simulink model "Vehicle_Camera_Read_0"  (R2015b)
settings: Solver=FixedStepDiscrete  StartTime=0.0  StopTime=inf  FixedStep=0.02  RelTol=1e-3
InitFcn:
  | Step_Size=0.02;
  | Speed_Steering_Right_Tire = [0 0 0.5 1 1 0.8 0.3 0 0];
  | Speed_Steering_Left_Tire=Speed_Steering_Right_Tire(end:-1:1);
  | Speed_Steering_Speed_Vector=4.*[-16 -15 -10 -5 0 5 10 15 16 ];
  | %plot(Speed_Steering_Speed_Vector,Speed_Steering_Right_Tire,'b',Speed_Steering_Speed_Vector,Speed_Steering_Left_Tire,'r');
  | 
  | Steering_Dead_Zone = 5;
libraries: frdmtfcshieldlib x4, Autonomous_Vehicle_Competition x1, frdmkl25zlib x1

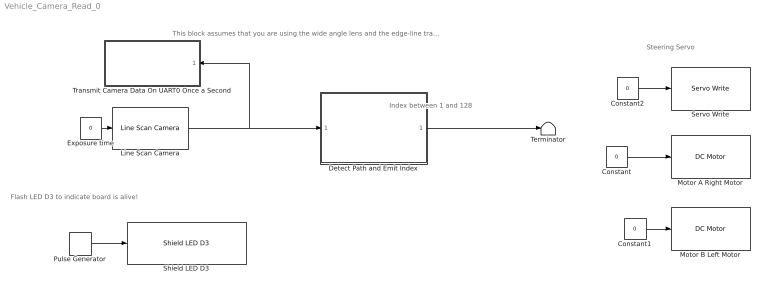
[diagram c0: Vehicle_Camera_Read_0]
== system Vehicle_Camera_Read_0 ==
  note: This block assumes that you are using the wide angle lens and the edge-line track.
  note: Steering Servo
  note: Index between 1 and 128
  note: Flash LED D3 to indicate board is alive!
  Constant : Constant  Value=0
  Constant1 : Constant  Value=0
  Constant2 : Constant  Value=0
  Detect Path and Emit Index : MATLAB Function  TreatAsAtomicUnit=on
  Exposure time : Constant  Value=0
  Line Scan Camera : frdmtfcshieldlib/Line Scan Camera  CameraHeader=0  SampleTime=.02
  Motor A Right Motor : frdmtfcshieldlib/DC Motor  WhichMotor=A
  Motor B Left Motor : frdmtfcshieldlib/DC Motor  WhichMotor=B
  Pulse Generator : DiscretePulseGenerator  PulseType=Time based  Period=1  PulseWidth=50
  Servo Write : frdmtfcshieldlib/Servo Write  WhichServo=0  minAngle=-90  maxAngle=90
  Shield LED D3 : Autonomous_Vehicle_Competition/Shield LED D3
  Terminator : Terminator
  Transmit Camera Data On UART0 Once a Second : Subsystem  TreatAsAtomicUnit=on  SystemSampleTime=.26
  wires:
  Pulse Generator/1 -> Shield LED D3/1
  Exposure time/1 -> Line Scan Camera/1
  Line Scan Camera/1 -> Transmit Camera Data On UART0 Once a Second/1(In1), Detect Path and Emit Index/1(Linescan_Data)
  Detect Path and Emit Index/1(centerIdx) -> Terminator/1
  Constant/1 -> Motor A Right Motor/1
  Constant1/1 -> Motor B Left Motor/1
  Constant2/1 -> Servo Write/1

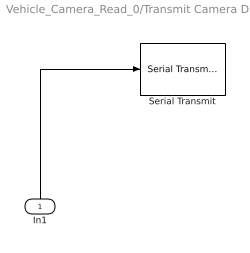
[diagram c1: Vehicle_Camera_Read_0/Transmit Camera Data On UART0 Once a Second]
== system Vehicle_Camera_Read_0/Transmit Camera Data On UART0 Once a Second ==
  In1 : Inport
  Serial Transmit : frdmkl25zlib/Serial Transmit  uart=UART0  sendmode=printf
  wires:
  In1/1 -> Serial Transmit/1

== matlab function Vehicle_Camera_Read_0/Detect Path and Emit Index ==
function centerIdx = CenterIdx(Linescan_Data)
% function centerIdx = CenterIdx(Linescan_Data)
% This function finds the current position of the track's
% center. 

%%---------------------------------------------------------------------------------------------
% The lines below are also inside  file "Full_High_School_Model_0_View_Camera.m"
% This m-file will display the camera data and also the edges and center of
% the track using the same algorithm the vehicle uses. If you modify the
% lines below, you must also modify the same lines in file
% "Full_High_School_Model_0_View_Camera.m".
% 

First_Edge=single(1);
Second_Edge=single(128);

% Calculate the threshold as 75% of the mean value of the bright section of
% the track.
Threshold=0.75*mean(Linescan_Data(40:80));

%Find the First Edge
for i=64:-1:2
    if Linescan_Data(i)<Threshold;
        First_Edge=single(i);
        break;
    end
end

% Find the Second Edge
for i=64:1:127
    if Linescan_Data(i)<Threshold;
        Second_Edge=single(i);
        break;
    end
end

% If the edge indices are valid, then calculate the 
% center as the average of the two edge indices.
if First_Edge>1 && Second_Edge<128
    centerIdx=(Second_Edge+First_Edge)/2;
else
    centerIdx=single(255);
end

%Paste changes to the lines above in inside  file "Full_High_School_Model_0_View_Camera.m"
%----------------------------------------------------------------------------------------------------------


%%end  minimum finding algorithm

end
